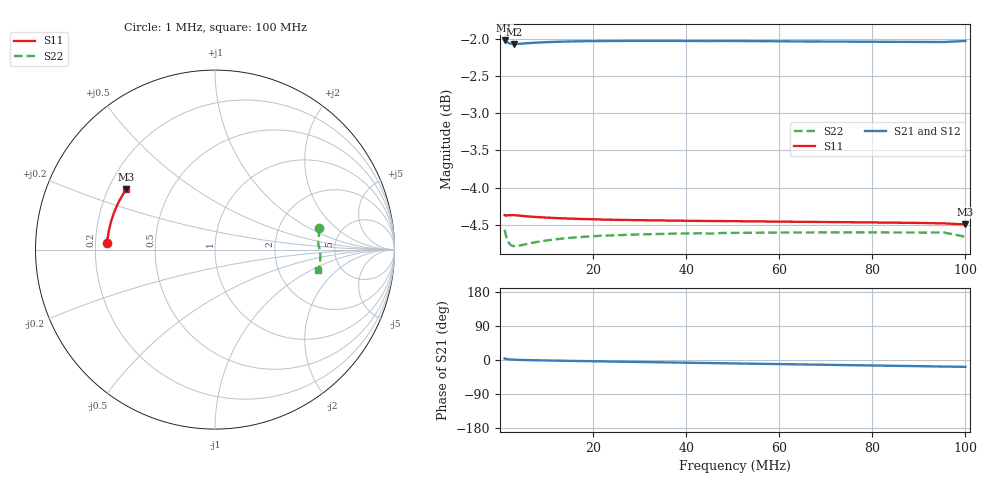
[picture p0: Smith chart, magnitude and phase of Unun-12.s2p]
! ListType=Log
!!Unun 12.5
# MHZ S RI R 50
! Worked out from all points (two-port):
!   100 points, 1 MHz to 100 MHz, reference 50 ohm
!   highest |S21| = -2.02 dB at 1 MHz (marker M1); lowest = -2.1 dB at 3.054 MHz (marker M2)
!   |S21| within 3 dB of the highest: start of sweep to end of sweep
!   lowest |S11| = -4.5 dB at 100 MHz (marker M3), VSWR 3.95, Z = 13.8 + j14.3 ohm
!   |S11| at or under -10 dB: nowhere
!   |S22| runs from -4.8 to -4.6 dB; largest |S21 - S12| = 0.0048
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1  -0.604 0.0342  0.79 0.0574  0.7897 0.0573  0.5793 0.1193
1.149757  -0.6038 0.0303  0.7903 0.048  0.79 0.048  0.5798 0.1012
1.321941  -0.6038 0.0272  0.79 0.04  0.7897 0.04  0.5794 0.086
1.519911  -0.604 0.0248  0.7894 0.0333  0.7891 0.0333  0.5783 0.0733
1.747528  -0.6043 0.0231  0.7888 0.0276  0.7885 0.0276  0.5772 0.0629
2.009233  -0.6044 0.0221  0.7883 0.0228  0.7881 0.0228  0.5763 0.0544
2.31013  -0.6045 0.0215  0.788 0.0186  0.7877 0.0186  0.5757 0.0473
2.656088  -0.6045 0.0214  0.7877 0.015  0.7875 0.0149  0.5754 0.0414
3.053856  -0.6044 0.0217  0.7877 0.0116  0.7874 0.0116  0.5754 0.0363
3.853529  -0.604 0.0231  0.7879 0.00638  0.7876 0.00638  0.576 0.0292
4.641589  -0.6036 0.025  0.7882 0.00231  0.788 0.00234  0.5769 0.0243
5.59081  -0.6032 0.0276  0.7886 -0.00182  0.7884 -0.00179  0.5779 0.0198
7.390722  -0.6023 0.033  0.7892 -0.00856  0.789 -0.00854  0.5797 0.0136
11.76812  -0.6003 0.0475  0.7901 -0.0225  0.7899 -0.0224  0.5826 0.00327
17.8865  -0.5973 0.0684  0.7901 -0.0399  0.79 -0.0398  0.5848 -0.0074
34.30469  -0.5867 0.1252  0.7871 -0.0834  0.7874 -0.0836  0.5867 -0.0305
45.34879  -0.5768 0.1627  0.7835 -0.1115  0.7833 -0.1126  0.5861 -0.0449
52.14008  -0.5696 0.1858  0.7808 -0.1289  0.7815 -0.1297  0.5862 -0.0532
68.92612  -0.548 0.2406  0.7722 -0.1705  0.773 -0.1723  0.5842 -0.0741
86.9749  -0.519 0.2965  0.7607 -0.2144  0.7611 -0.2172  0.5809 -0.0965
95.45485  -0.5031 0.3217  0.7545 -0.235  0.7544 -0.238  0.579 -0.1071
100  -0.4932 0.3349  0.7523 -0.2459  0.7489 -0.2492  0.5735 -0.1152
